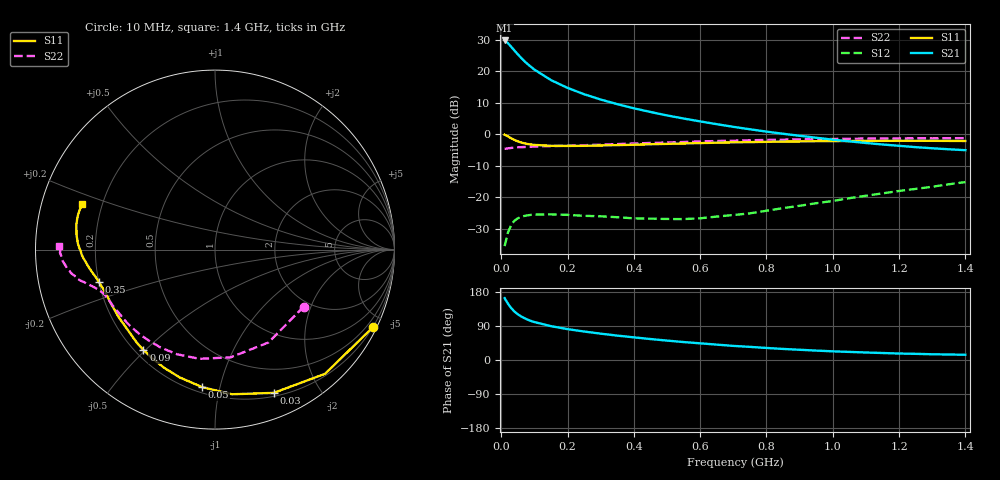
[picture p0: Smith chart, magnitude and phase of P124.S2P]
! Date: Tue Aug 08 08:19:31 1995
# MHZ  S  MA  R  50.0000
!  POLYFET RF DEVICES
!  P124
!  S PARAMETERS
!  VDS=12.5V, IDQ=400mA
!FREQ  S11MAG S11ANG S21MAG S21ANG S12MAG S12ANG S22MAG S22ANG
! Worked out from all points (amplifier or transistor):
!   36 points, 10 MHz to 1.4 GHz, reference 50 ohm
!   highest |S21| = 29.7 dB at 10 MHz (marker M1)
!   |S21| within 3 dB of that: start of sweep to 38.07 MHz
!   unconditionally stable (mu >= 1): 503.9 MHz to 779.5 MHz
!   at 70 MHz: K = 0.14, MSG = 24.5 dB, |S12| = -25.9 dB
!   at 550 MHz: K = 1.07, MAG = 14.4 dB, |S12| = -26.9 dB
!   at 1.4 GHz: K = 0.57, MSG = 5.1 dB, |S12| = -15.2 dB
!   S11 on the Smith chart (normalised r, x): 10 MHz: 0.19, -4.30; 30 MHz: 0.23, -1.46; 50 MHz: 0.23, -0.88; 90 MHz: 0.23, -0.49; 350 MHz: 0.20, -0.13; 1.4 GHz: 0.13, +0.16
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10  0.9808 -26.1  30.56 163.2  0.01687 72.8  0.5877 -32.7
20  0.9246 -48.4  27.68 148.7  0.0277 60.4  0.597 -60.1
30  0.8627 -67.7  24.26 136.9  0.03658 49.4  0.6066 -81.7
40  0.8115 -83.3  21.05 127.6  0.04298 41.7  0.6146 -98.1
50  0.7699 -95.3  18.39 120.5  0.04671 34.8  0.6204 -110.1
60  0.7388 -105.4  16.15 114.9  0.04899 30.0  0.6239 -119.2
70  0.7168 -113.3  14.3 110.2  0.05092 27.2  0.627 -126.3
80  0.6989 -120.1  12.84 106.3  0.05199 23.9  0.6313 -131.8
90  0.6871 -125.5  11.61 103.0  0.05285 21.3  0.6342 -136.2
100  0.6771 -130.1  10.54 100.0  0.05332 19.6  0.6376 -140.0
150  0.6557 -145.1  7.194 89.3  0.05377 13.8  0.6485 -150.6
200  0.6529 -153.1  5.417 81.5  0.05284 11.6  0.6572 -155.8
250  0.6555 -158.2  4.296 75.1  0.05104 10.7  0.6696 -158.9
300  0.6634 -161.8  3.542 69.5  0.05015 11.6  0.6844 -160.8
350  0.6722 -164.6  2.995 64.3  0.04847 14.0  0.6978 -162.0
400  0.6815 -166.9  2.574 59.8  0.04652 16.2  0.7126 -163.3
500  0.7039 -170.9  1.985 51.2  0.04548 25.4  0.7397 -165.1
600  0.7241 -174.6  1.595 44.0  0.04663 36.0  0.7695 -167.0
750  0.7491 -179.5  1.198 34.7  0.0558 49.8  0.8025 -169.9
950  0.7752 174.2  0.8795 24.8  0.08083 60.1  0.835 -173.6
1200  0.7871 167.0  0.6555 17.1  0.1264 61.7  0.8594 -178.1
1400  0.7807 161.1  0.5588 13.9  0.1746 57.9  0.8669 178.7
